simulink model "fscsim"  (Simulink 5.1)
settings: Solver=ode45  SolverMode=SingleTasking  StartTime=0.0  StopTime=20e-3  MaxStep=Ts/10  RelTol=1e-3  AbsTol=1e-6
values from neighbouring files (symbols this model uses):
  Ts = PlantDataSeek.Ts    [seekdemo.m]    (also in HDDBenchPlot.m = PlantData.Ts; hdd_plantparam.m = 3.78787878788e-05; SetDistParam.m = PlantData.Ts; SetFlutterDist.m = PlantData.Ts)
undefined symbols (not defined in the file or in its folder): apf, bpf, cpf, dpf

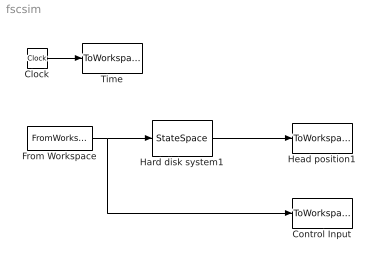
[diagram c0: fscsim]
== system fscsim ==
  Clock : Clock
  Control Input : ToWorkspace  VariableName=us  SampleTime=Ts/10  SaveFormat=Array
  From Workspace : FromWorkspace  VariableName=[tr' U]  SampleTime=Ts  Interpolate=off  OutputAfterFinalValue=Holding final value
  Hard disk system1 : StateSpace  A=apf  B=bpf  C=cpf  D=dpf
  Head position1 : ToWorkspace  VariableName=ys  SampleTime=Ts/10  SaveFormat=Array
  Time : ToWorkspace  VariableName=ts  SampleTime=Ts/10  SaveFormat=Array
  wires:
  Clock/1 -> Time/1
  Hard disk system1/1 -> Head position1/1
  From Workspace/1 -> Hard disk system1/1, Control Input/1
